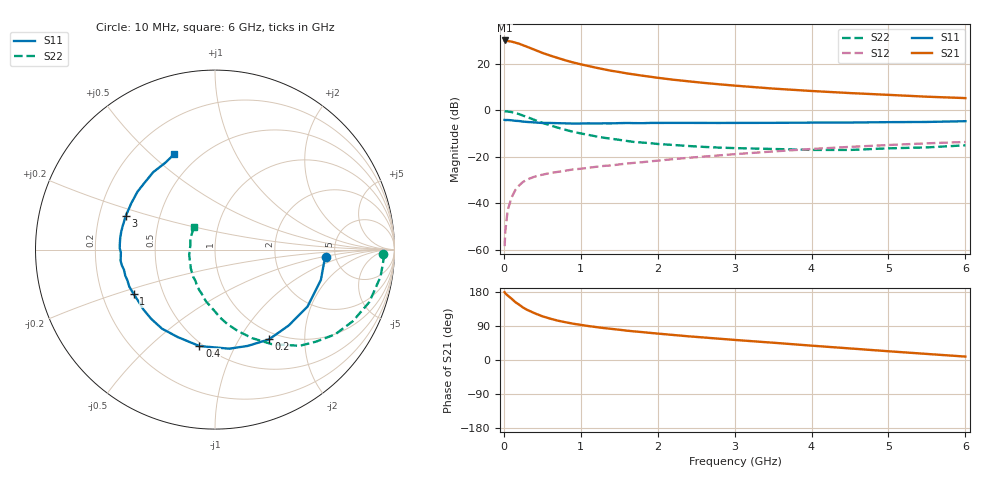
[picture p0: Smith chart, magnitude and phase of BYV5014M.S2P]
! SIEMENS Small Signal Semiconductors
! BFY420
! Si NPN RF SIEGET Grounded Emitter Transistor in MICRO-X
! VCE = 0.5 V  IC = 14 mA
! Common Emitter S-Parameters:  October  1996
# GHz  S  MA  R  50
!  f  S11  S21  S12  S22
! GHz  MAG  ANG  MAG  ANG  MAG  ANG  MAG  ANG
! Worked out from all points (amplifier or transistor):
!   36 points, 10 MHz to 6 GHz, reference 50 ohm
!   highest |S21| = 29.9 dB at 10 MHz (marker M1)
!   |S21| within 3 dB of that: start of sweep to 323.1 MHz
!   unconditionally stable (mu >= 1): 1.92 GHz to end of sweep
!   at 250 MHz: K = 0.26, MSG = 29.3 dB, |S12| = -30.8 dB
!   at 1.4 GHz: K = 0.90, MSG = 20.3 dB, |S12| = -23.7 dB
!   at 6 GHz: K = 1.12, MAG = 7.3 dB, |S12| = -13.7 dB
!   S11 on the Smith chart (normalised r, x): 10 MHz: 4.17, -0.52; 200 MHz: 0.89, -1.35; 400 MHz: 0.48, -0.73; 1 GHz: 0.34, -0.23; 3 GHz: 0.32, +0.17; 6 GHz: 0.37, +0.60
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0.01  0.618 -3.6  31.32 178.9  0.0012 93.4  0.9388 -1.6
0.02  0.6119 -6.7  31.23 175.7  0.0026 87.3  0.9407 -3.5
0.05  0.6137 -16.0  30.45 170.2  0.0071 80.6  0.9346 -9.3
0.1  0.6054 -31.6  29.63 161.9  0.0133 76.8  0.9081 -18.8
0.15  0.5894 -45.9  28.07 152.6  0.0193 69.8  0.8652 -27.5
0.2  0.5836 -59.0  26.59 145.8  0.0243 65.4  0.8192 -35.2
0.25  0.5668 -71.2  24.73 138.5  0.0288 60.5  0.761 -42.4
0.3  0.5577 -81.8  22.95 132.7  0.0322 57.8  0.7145 -48.6
0.4  0.5444 -99.2  19.77 123.4  0.0373 52.4  0.6146 -59.0
0.5  0.5297 -113.1  16.96 115.4  0.0411 49.0  0.5344 -67.3
0.6  0.5304 -123.8  14.88 109.3  0.0445 47.2  0.4721 -74.2
0.7  0.5246 -132.8  13.2 103.9  0.0472 45.9  0.4211 -80.5
0.9  0.5148 -146.0  10.56 95.8  0.0533 44.8  0.3423 -90.4
1  0.5163 -151.4  9.628 92.7  0.0551 44.4  0.3161 -94.8
1.1  0.5203 -156.6  8.854 89.6  0.0578 44.7  0.2943 -99.5
1.6  0.5296 -173.2  6.141 77.4  0.0713 44.9  0.2182 -118.3
2.2  0.532 173.3  4.502 66.1  0.0885 44.2  0.1789 -136.4
3  0.5313 159.3  3.36 53.0  0.1133 40.8  0.153 -156.6
3.5  0.5332 151.0  2.901 45.6  0.1297 37.8  0.1466 -168.7
4.5  0.5415 136.1  2.324 30.5  0.1626 29.4  0.1396 168.5
5.5  0.5574 119.9  1.942 16.0  0.1937 19.8  0.1584 143.0
6  0.5785 113.0  1.813 9.0  0.2072 14.7  0.1756 133.0
